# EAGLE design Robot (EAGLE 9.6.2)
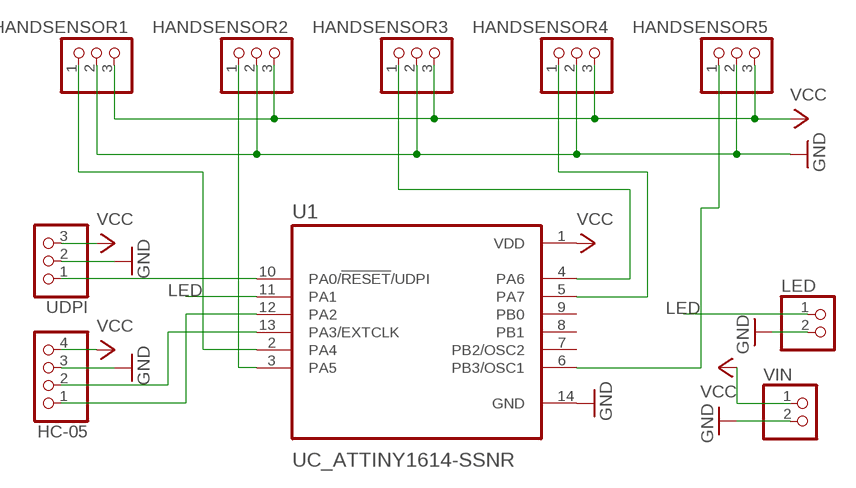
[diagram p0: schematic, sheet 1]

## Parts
HANDSENSOR1  PINHD-1X3  [1X03]
HANDSENSOR2  PINHD-1X3  [1X03]
HANDSENSOR3  PINHD-1X3  [1X03]
HANDSENSOR4  PINHD-1X3  [1X03]
HANDSENSOR5  PINHD-1X3  [1X03]
HC-05  PINHD-1X4  [1X04]
LED  PINHD-1X2  [1X02]
U1  UC_ATTINY1614-SSNR  [SOIC127P600X175-14N]
UDPI  PINHD-1X3  [1X03]
VIN  PINHD-1X2  [1X02]

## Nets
GND: HANDSENSOR1.2 HANDSENSOR2.2 HANDSENSOR3.2 HANDSENSOR4.2 HANDSENSOR5.2 HC-05.3 LED.2 U1.14(GND) UDPI.2 VIN.2
LED: LED.1 U1.11(PA1)
N$1: U1.10(PA0/!RESET!/UDPI) UDPI.1
N$2: HC-05.1 U1.12(PA2)
N$3: HC-05.2 U1.13(PA3/EXTCLK)
N$4: HANDSENSOR1.1 U1.2(PA4)
N$5: HANDSENSOR2.1 U1.3(PA5)
N$6: HANDSENSOR3.1 U1.4(PA6)
N$7: HANDSENSOR4.1 U1.5(PA7)
N$8: HANDSENSOR5.1 U1.6(PB3/OSC1)
VCC: HANDSENSOR1.3 HANDSENSOR2.3 HANDSENSOR3.3 HANDSENSOR4.3 HANDSENSOR5.3 HC-05.4 U1.1(VDD) UDPI.3 VIN.1
Unconnected: U1.7(PB2/OSC2) U1.8(PB1) U1.9(PB0)

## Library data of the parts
HANDSENSOR1-HANDSENSOR5 UDPI = pinhead:PINHD-1X3: PIN HEADER
HC-05 = pinhead:PINHD-1X4: PIN HEADER
LED VIN = pinhead:PINHD-1X2: PIN HEADER
U1 = fab:UC_ATTINY1614-SSNR: 20MHz, SOIC, 85C, Green, 14 SOIC .150in T/R Check prices; AVAILABILITY: In Stock; DESCRIPTION: AVR tinyAVR™ 1, Functional Safety (FuSa) Microcontroller IC 8-Bit 20MHz 16KB (16K x 8) FLASH 14-SOIC; MF: Microchip Technology; MP: ATTINY1614-SSNR; PACKAGE: None; PRICE: None; PURCHASE-URL: https://pricing.snapeda.com/search/part/ATTINY1614-SSNR/?ref=eda

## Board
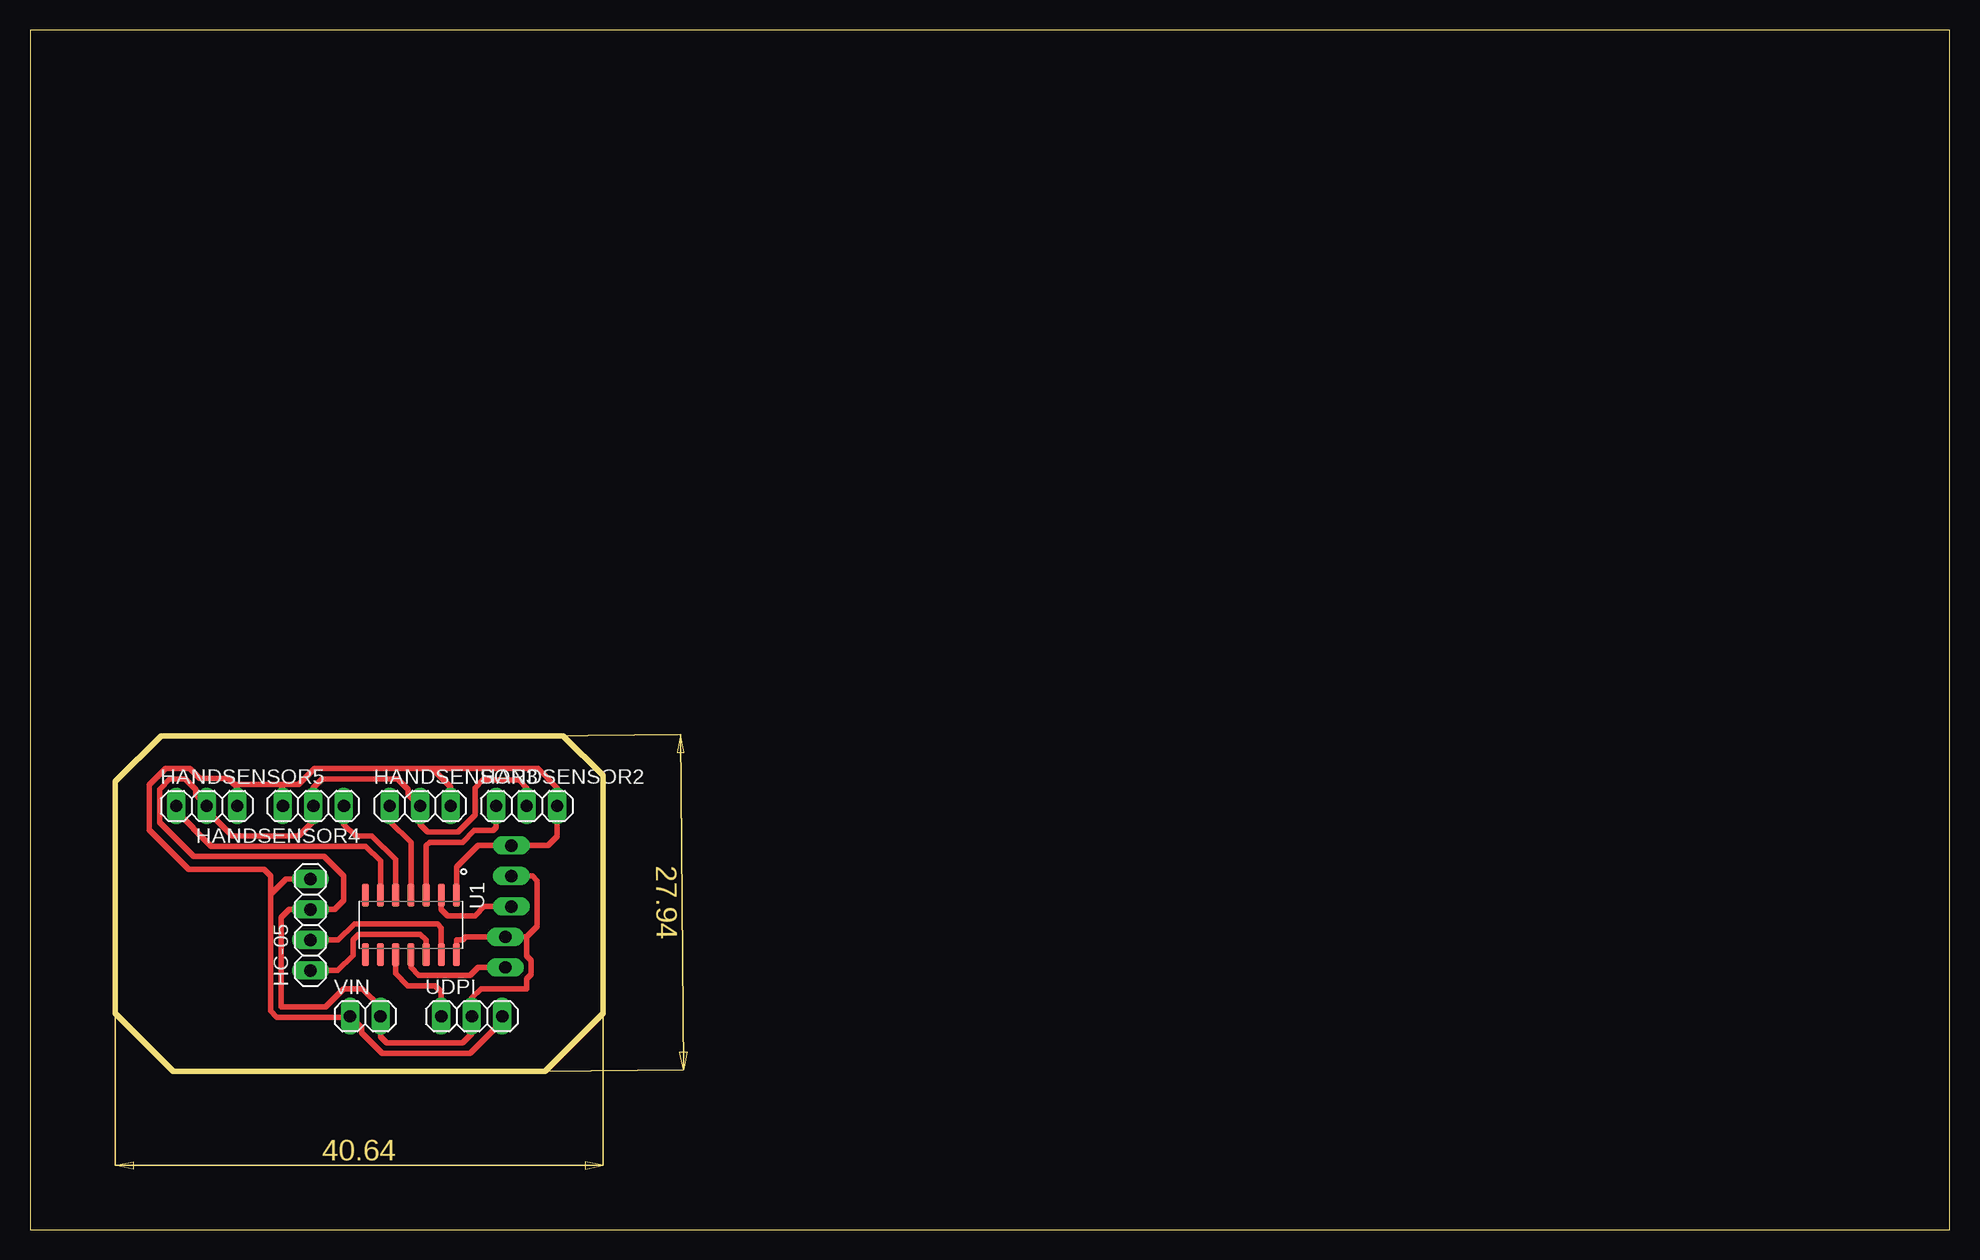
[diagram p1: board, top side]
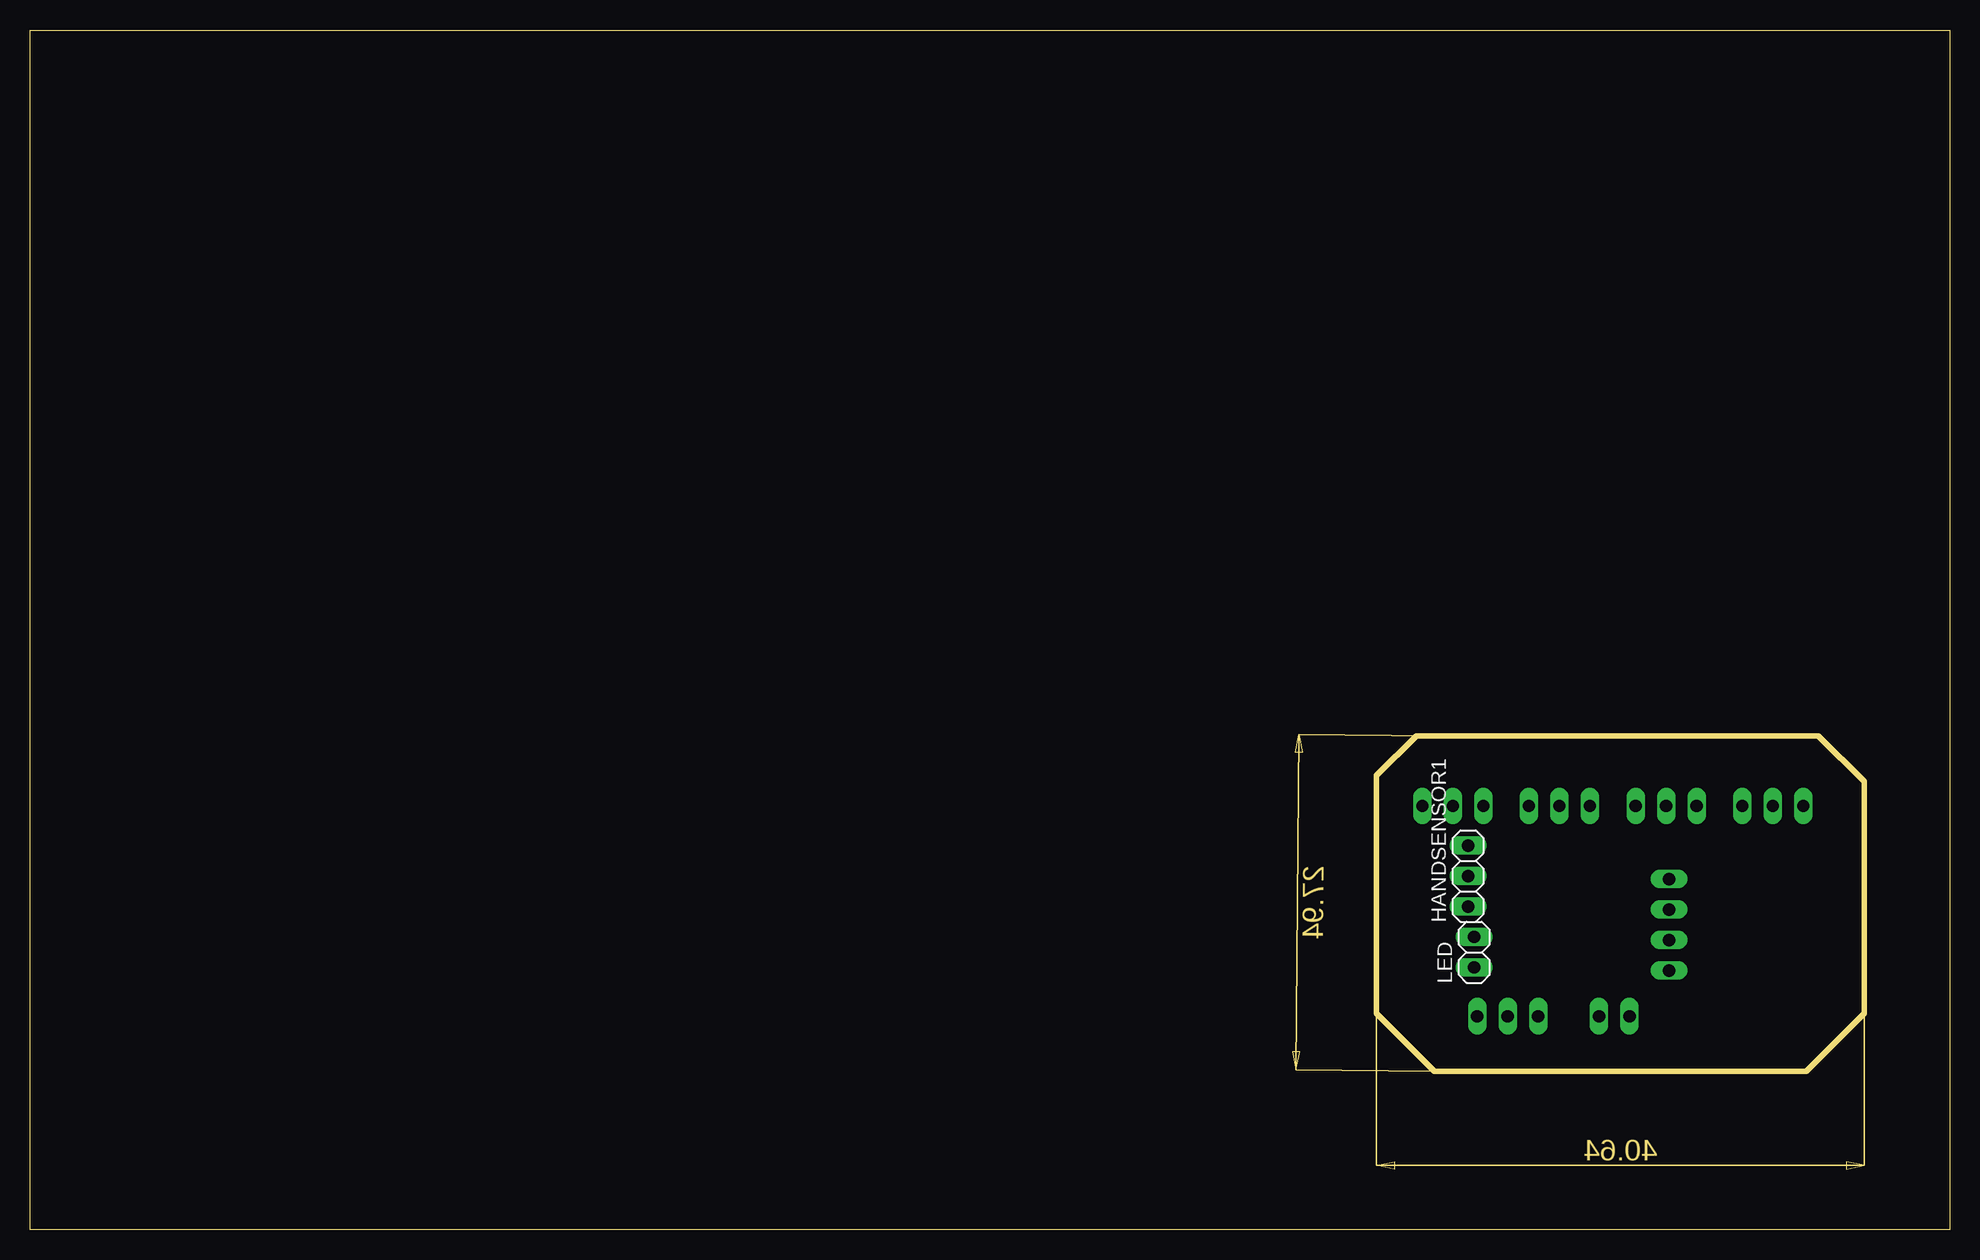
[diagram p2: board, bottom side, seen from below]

Size 160 x 100 mm. Coordinates in mm from the lower left corner, seen from the top.
Outline: 0,0 160,0 160,100 0,100 0,0
Copper layers (1*16): Top 0.035mm / dielectric 1.5mm / Bottom 0.035mm
Design rules "default *": minimum track width 18mil, minimum drill 0.35mm, track to track 16mil, track to pad 16mil, pad to pad 16mil, via to via 12mil, smd to smd 10mil, copper to edge 40mil, drill to drill 6mil, minimum pad ring 10mil, minimum via ring 8mil, stop-mask expansion 4mil, vias tented up to drill 0mil, thermal gap 10mil
Milling: area 7.1,5 to 8.6,5.6; area 46.3,5 to 47.8,5.6; area 24,5.7 to 30.9,7.5; area 54.2,13.3 to 54.8,14.8; area 53.9,39.8 to 54.5,41.3; area 52.1,23.8 to 54,30.7; 16 lines

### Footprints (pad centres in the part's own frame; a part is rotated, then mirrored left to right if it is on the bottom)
1X03 = drill 1.016 long: 1 -2.54,0; 2 0,0; 3 2.54,0
1X04 = drill 1.016 long: 1 -3.81,0; 2 -1.27,0; 3 1.27,0; 4 3.81,0
1X02 = drill 1.016 long: 1 -1.27,0; 2 1.27,0
SOIC127P600X175-14N = smd 1.95 x 0.59: 1 -2.48,3.81; 2 -2.48,2.54; 3 -2.48,1.27; 4 -2.48,0; 5 -2.48,-1.27; 6 -2.48,-2.54; 7 -2.48,-3.81; 8 2.48,-3.81; 9 2.48,-2.54; 10 2.48,-1.27; 11 2.48,0; 12 2.48,1.27; 13 2.48,2.54; 14 2.48,3.81

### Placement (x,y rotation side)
HANDSENSOR1  40.13,29.46 90 bottom
HANDSENSOR2  41.4,35.31 0 top
HANDSENSOR3  32.51,35.31 0 top
HANDSENSOR4  23.62,35.31 180 top
HANDSENSOR5  14.73,35.31 0 top
HC-05  23.37,25.4 90 top
LED  39.62,23.11 90 bottom
U1  31.75,25.4 270 top
UDPI  36.83,17.78 0 top
VIN  27.94,17.78 0 top

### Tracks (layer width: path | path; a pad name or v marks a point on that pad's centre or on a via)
GND
  Top 0.457: U1.14 35.56,24.13 36.07,24.13 36.32,24.38 LED.2 41.4,24.38 | HANDSENSOR2.2 41.4,36.83 40.77,37.47 37.72,37.47 37.08,36.83 37.08,34.54 35.69,33.15 33.15,33.15 32.51,33.78 HANDSENSOR3.2 32.38,35.41 31.52,36.27 31.52,36.7 30.66,37.57 24.36,37.57 23.62,36.83 HANDSENSOR4.2 23.62,34.04 22.4,32.82 16.84,32.82 15.11,34.54 15.11,34.98 HANDSENSOR5.2 14.68,35.41 13.82,36.27 13.82,36.7 12.95,37.57 11.66,37.57 10.79,36.7 10.79,33.93 13.64,31.09 24.54,31.09 26.16,29.46 26.16,27.43 25.4,26.67 HC-05.3 21.59,26.67 20.93,26.01 20.93,18.57 24.66,18.57 26.16,20.07 27.69,20.07 29.21,18.54 VIN.2 29.21,16.05 29.72,15.54 36.07,15.54 36.83,16.31 UDPI.2 36.83,19.3 37.59,20.07 41.4,20.07 41.4,20.88 41.78,21.27 41.78,22.42 41.4,22.8 41.4,24.38 | 41.4,24.38 42.29,25.27 42.29,29.08 41.91,29.46 HANDSENSOR1.2
LED
  Top 0.457: U1.11 31.75,21.84 32.41,21.18 36.68,21.18 37.34,21.84 LED.1
N$1
  Top 0.457: U1.10 30.48,21.34 31.5,20.32 33.78,20.32 34.29,19.81 UDPI.1
N$2
  Top 0.457: U1.12 33.02,24.13 32.54,24.61 27.41,24.61 26.92,24.13 26.92,22.86 25.65,21.59 HC-05.1
N$3
  Top 0.457: U1.13 34.29,25.15 33.96,25.48 27.05,25.48 25.7,24.13 HC-05.2
N$4
  Top 0.457: U1.2 34.29,26.67 34.8,26.16 37.08,26.16 37.85,26.92 HANDSENSOR1.1
N$5
  Top 0.457: U1.3 33.02,32 33.3,32.28 36.05,32.28 37.03,33.27 38.61,33.27 38.86,33.53 HANDSENSOR2.1
N$6
  Top 0.457: HANDSENSOR3.1 29.97,34.04 31.75,32.26 U1.4
N$7
  Top 0.457: U1.5 30.48,30.84 28.5,32.82 27.13,32.82 26.16,33.78 HANDSENSOR4.1
N$8
  Top 0.457: HANDSENSOR5.1 12.09,34.98 15.11,31.95 27.99,31.95 29.21,30.73 U1.6
VCC
  Top 0.457: UDPI.3 39.37,17.35 36.7,14.68 29.36,14.68 27.64,16.41 27.64,16.84 26.77,17.7 VIN.1 26.34,17.7 20.57,17.7 20.07,18.21 20.07,27.94 | 17.02,37.08 16.51,37.59 14.15,37.59 13.31,38.43 11.3,38.43 9.93,37.06 9.93,33.32 13.23,30.02 19.51,30.02 20.07,29.46 20.07,27.94 | 17.02,37.08 17.27,36.83 HANDSENSOR5.3 | 17.02,37.08 20.83,37.08 | 20.83,37.08 21.08,36.83 HANDSENSOR4.3 | 20.83,37.08 22.4,37.08 23.75,38.43 33.53,38.43 | 33.53,38.43 35.05,36.91 HANDSENSOR3.3 | U1.1 35.56,30.23 37.34,32 HANDSENSOR1.3 43.18,32 43.94,32.77 HANDSENSOR2.3 43.94,36.83 42.34,38.43 33.53,38.43 | 20.07,27.94 21.34,29.21 HC-05.4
